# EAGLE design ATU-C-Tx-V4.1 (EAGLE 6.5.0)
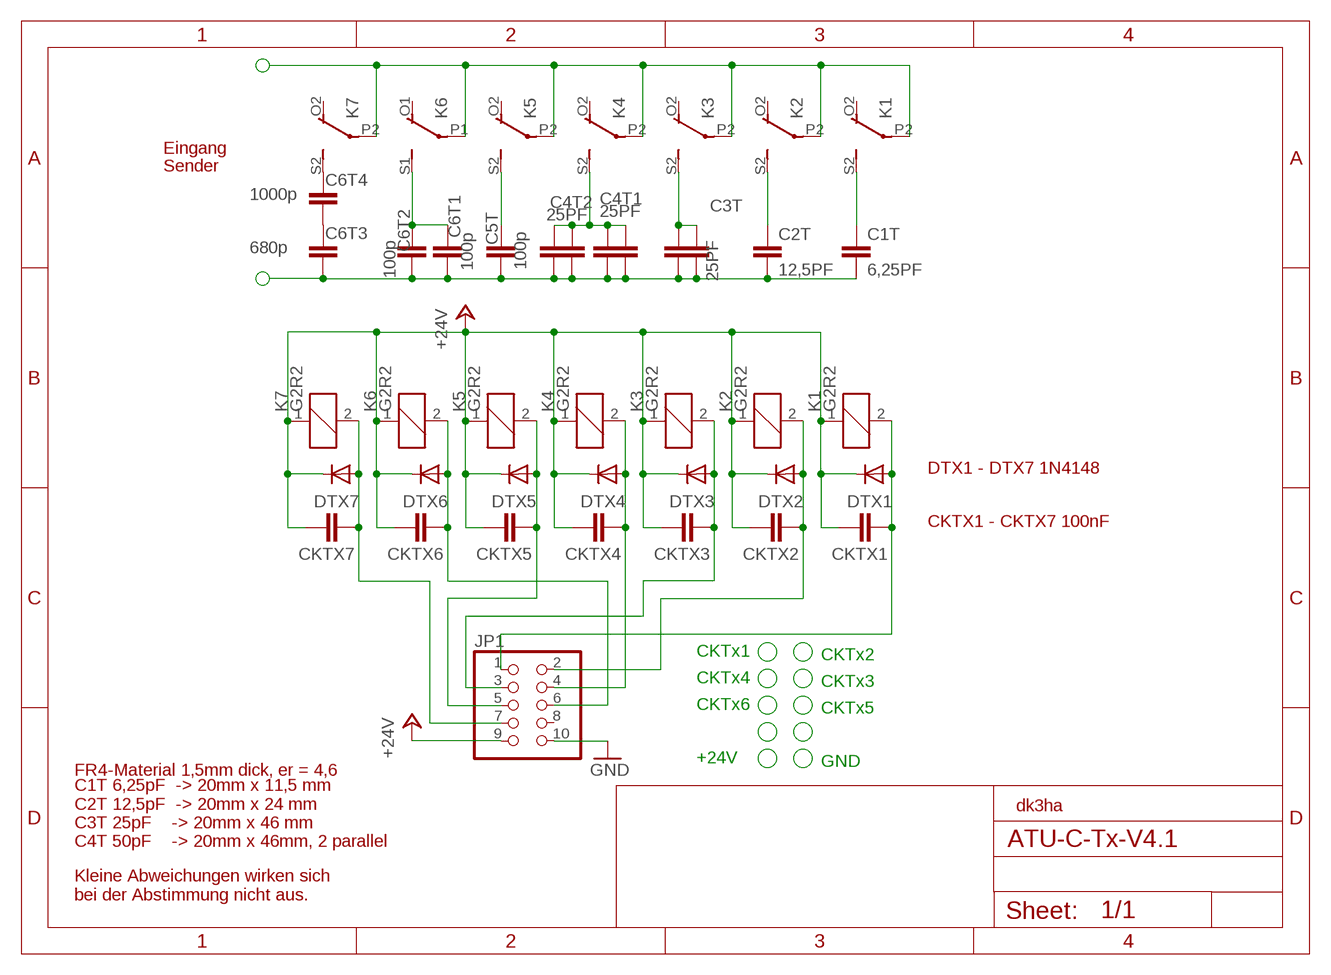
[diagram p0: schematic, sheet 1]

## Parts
C1T  6,25PF  6,25PF-CU-DS-ER4,6-D1,5  [6,25-ERA4,6-DS-1,5]
C2T  12,5PF  12,5PF-CU-DS-ER4,6-D1,5  [12.5-ER4.6-DS-1,5]
C3T  25PF  25PF-CU-DS-ER4,6-D-1,5  [25PF_ER4.6-DS-1,5]
C4T1  25PF  25PF-CU-DS-ER4,6-D-1,5  [25PF_ER4.6-DS-1,5]
C4T2  25PF  25PF-CU-DS-ER4,6-D-1,5  [25PF_ER4.6-DS-1,5]
C5T  100p  C15/5  [C15B5]
C6T1  100p  C15/5  [C15B5]
C6T2  100p  C15/5  [C15B5]
C6T3  680p  C15/5  [C15B5]
C6T4  1000p  C15/5  [C15B5]
CKTX1  C-EUC1206  [C1206]
CKTX2  C-EUC1206  [C1206]
CKTX3  C-EUC1206  [C1206]
CKTX4  C-EUC1206  [C1206]
CKTX5  C-EUC1206  [C1206]
CKTX6  C-EUC1206  [C1206]
CKTX7  C-EUC1206  [C1206]
DTX1  DIODE-MINIMELF  [MINIMELF]
DTX2  DIODE-MINIMELF  [MINIMELF]
DTX3  DIODE-MINIMELF  [MINIMELF]
DTX4  DIODE-MINIMELF  [MINIMELF]
DTX5  DIODE-MINIMELF  [MINIMELF]
DTX6  DIODE-MINIMELF  [MINIMELF]
DTX7  DIODE-MINIMELF  [MINIMELF]
JP1  PINHD-2X5  [2X05]
K1  G2R2  [G2R2]
K2  G2R2  [G2R2]
K3  G2R2  [G2R2]
K4  G2R2  [G2R2]
K5  G2R2  [G2R2]
K6  G2R2  [G2R2]
K7  G2R2  [G2R2]

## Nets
+24V: CKTX1.2 CKTX2.2 CKTX3.2 CKTX4.2 CKTX5.2 CKTX6.2 CKTX7.2 DTX1.C DTX2.C DTX3.C DTX4.C DTX5.C DTX6.C DTX7.C JP1.9 K1.1 K2.1 K3.1 K4.1 K5.1 K6.1 K7.1
GND: JP1.10
LSP7: K1.P2(3:P) K2.P2(3:P) K3.P2(3:P) K4.P2(3:P) K5.P2(3:P) K6.P1(2:P) K7.P2(3:P)
LSP8: C1T.P$2 C2T.P$2 C3T.P$2 C3T.P$4 C4T1.P$2 C4T1.P$4 C4T2.P$2 C4T2.P$4 C5T.2 C6T1.2 C6T2.1 C6T3.1
N$1: CKTX4.1 DTX4.A JP1.4 K4.2
N$2: C4T1.P$1 C4T1.P$3 C4T2.P$1 C4T2.P$3 K4.S2(3:S)
N$3: C6T1.1 C6T2.2 K6.S1(2:S)
N$4: CKTX7.1 DTX7.A JP1.7 K7.2
N$5: C3T.P$1 C3T.P$3 K3.S2(3:S)
N$6: C2T.P$1 K2.S2(3:S)
N$7: C1T.P$1 K1.S2(3:S)
N$8: C5T.1 K5.S2(3:S)
N$9: C6T4.2 K7.S2(3:S)
N$10: C6T3.2 C6T4.1
N$E1: CKTX1.1 DTX1.A JP1.1 K1.2
N$E2: CKTX2.1 DTX2.A JP1.2 K2.2
N$E3: CKTX3.1 DTX3.A JP1.3 K3.2
N$E5: CKTX5.1 DTX5.A JP1.5 K5.2
N$E6: CKTX6.1 DTX6.A JP1.6 K6.2
Unconnected: JP1.8 K1.O1(2:O) K1.O2(3:O) K1.P1(2:P) K1.S1(2:S) K2.O1(2:O) K2.O2(3:O) K2.P1(2:P) K2.S1(2:S) K3.O1(2:O) K3.O2(3:O) K3.P1(2:P) K3.S1(2:S) K4.O1(2:O) K4.O2(3:O) K4.P1(2:P) K4.S1(2:S) K5.O1(2:O) K5.O2(3:O) K5.P1(2:P) K5.S1(2:S) K6.O1(2:O) K6.O2(3:O) K6.P2(3:P) K6.S2(3:S) K7.O1(2:O) K7.O2(3:O) K7.P1(2:P) K7.S1(2:S)

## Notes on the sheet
- Eingang
- Sender
- DTX1 - DTX7 1N4148
- CKTX1 - CKTX7 100nF
- CKTx1 | CKTx2
- CKTx4 | CKTx3
- CKTx6 | CKTx5
- +24V | GND
- FR4-Material 1,5mm dick, er = 4,6
- dk3ha
- C1T 6,25pF  -> 20mm x 11,5 mm
  C2T 12,5pF  -> 20mm x 24 mm
  C3T 25pF    -> 20mm x 46 mm
  C4T 50pF    -> 20mm x 46mm, 2 parallel
- Kleine Abweichungen wirken sich
  bei der Abstimmung nicht aus.

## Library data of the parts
C1T = dk3ha-2020:6,25PF-CU-DS-ER4,6-D1,5: C doppelseitig Cu, d=1,5mm, Epoxy er=4,6 (Bungard), 25 pF, Maße 18,7mm x 13mm
C2T = dk3ha-2020:12,5PF-CU-DS-ER4,6-D1,5: C doppelseitig Cu, d=1,5mm, Epoxy er=4,6 (Bungard), 25 pF, Maße 27,5mm x 18mm
C3T C4T1 C4T2 = dk3ha-2020:25PF-CU-DS-ER4,6-D-1,5: C doppelseitig Cu, d=1,5mm, Epoxy er=4,6 (Bungard), 25 pF, Maße 49,4mm x 18mm
C5T C6T1-C6T4 = capacitor-wima:C: CAPACITOR
CKTX1-CKTX7 = rcl:C-EU: CAPACITOR, European symbol
DTX1-DTX7 = diode:DIODE-: DIODE
JP1 = pinhead+:PINHD-2X5: PIN HEADER
K1-K7 = relay:G2R2: RELAY 2 x switch, Omron; MF: OMRON COMPONENTS USA; MPN: G2R-2-DC6; OC_FARNELL: unknown; OC_NEWARK: 89C5317

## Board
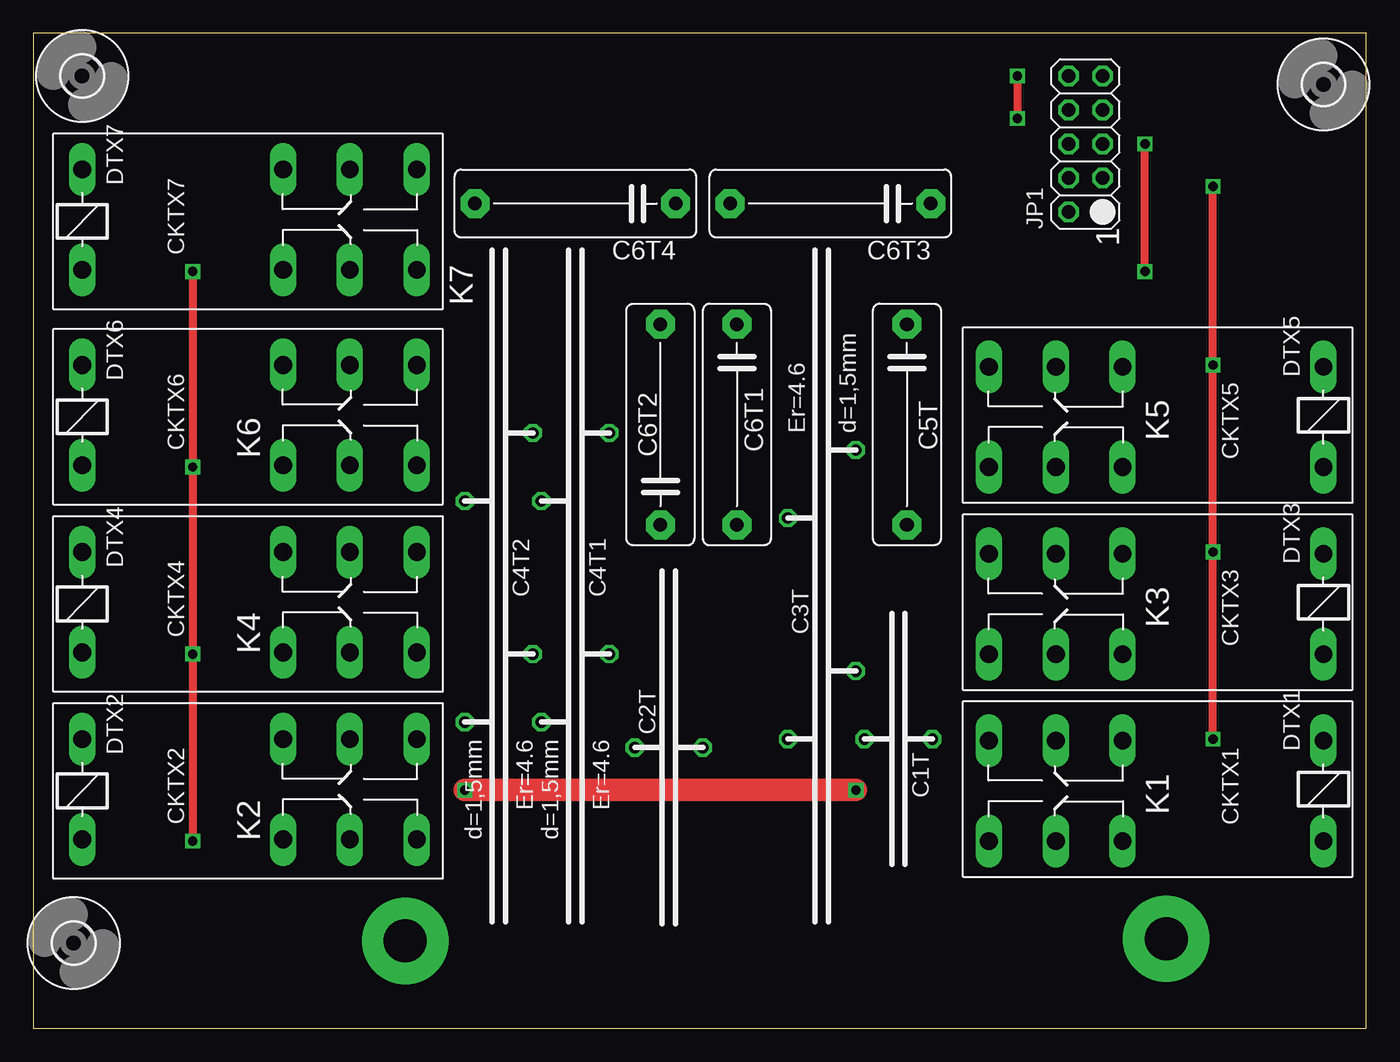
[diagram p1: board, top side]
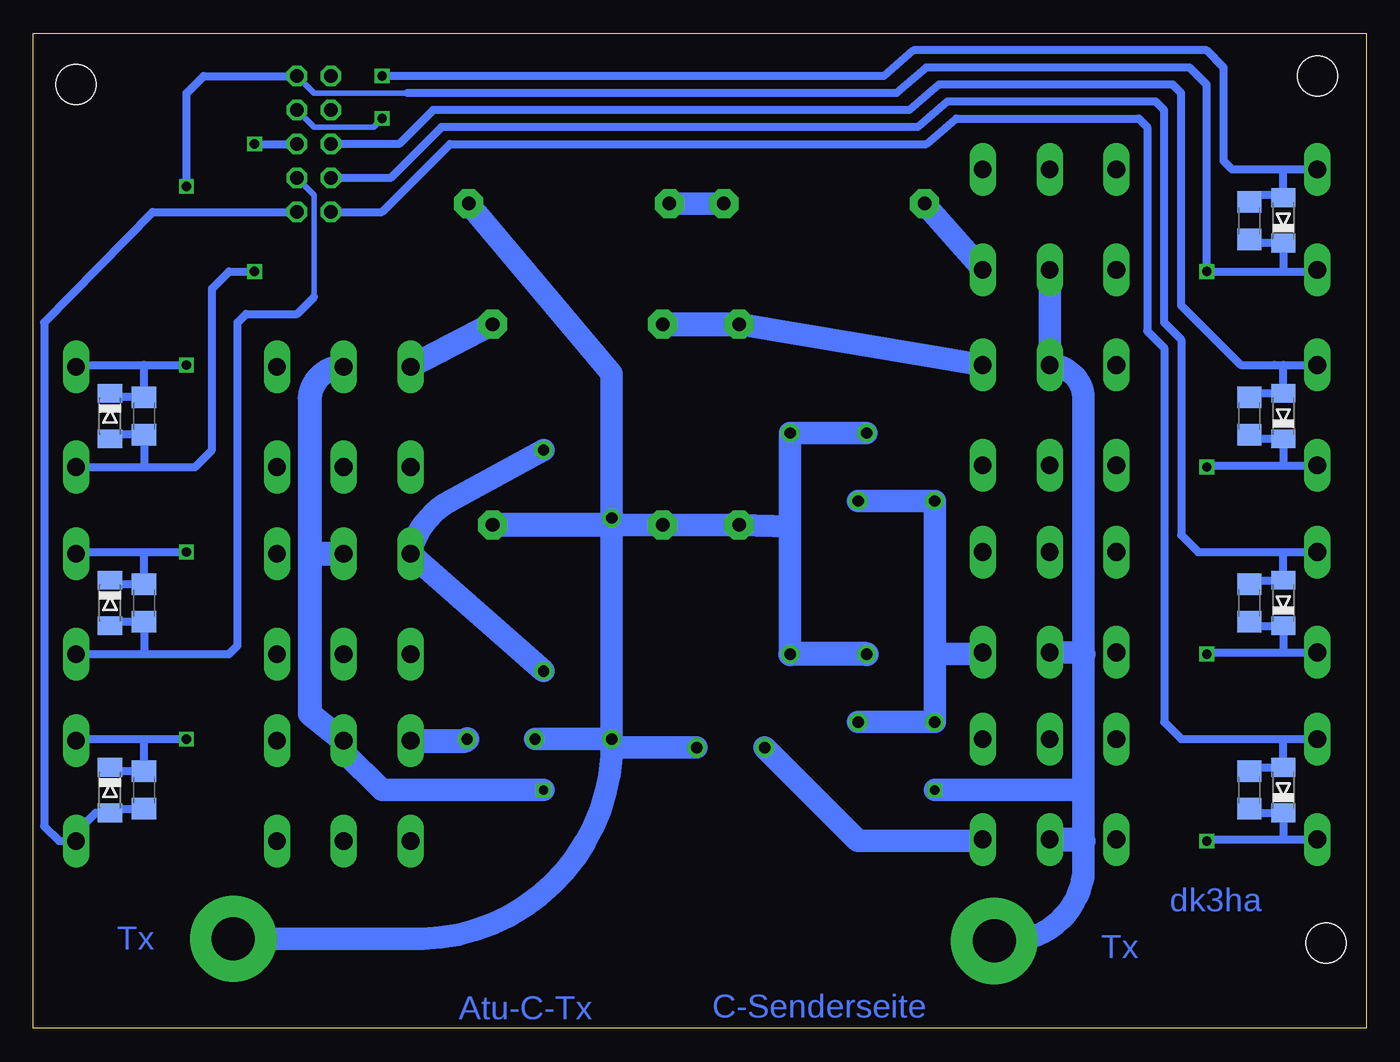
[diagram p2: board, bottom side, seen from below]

Size 99.52 x 74.3 mm. Coordinates in mm from the lower left corner, seen from the top.
Outline: 99.52,0 99.52,74.3 0,74.3 0,0 99.52,0
Copper layers (1*16): Top 0.035mm / dielectric 1.5mm / Bottom 0.035mm
Design rules "default": minimum track width 10mil, minimum drill 24mil, track to track 8mil, track to pad 8mil, pad to pad 8mil, via to via 8mil, smd to smd 8mil, copper to edge 40mil, drill to drill 8mil, minimum pad ring 10mil, minimum via ring 8mil, stop-mask expansion 4mil, vias tented up to drill 0mil, thermal gap 10mil

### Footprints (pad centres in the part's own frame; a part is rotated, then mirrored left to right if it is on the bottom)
6,25-ERA4,6-DS-1,5 = drill 0.85 octagon: P$1 -2.54,0; P$2 2.54,0
12.5-ER4.6-DS-1,5 = drill 0.85 octagon: P$1 -2.54,0; P$2 2.54,0
25PF_ER4.6-DS-1,5 = drill 0.85 pad 1.27 octagon: P$1 0,0; P$2 -5.08,-5.08 | drill 0.85 octagon: P$3 0,-16.51; P$4 -5.08,-21.59
C15B5 = drill 1.016 pad 2.159 octagon: 1 -7.493,0; 2 7.493,0
C1206 = smd 1.6 x 1.8: 1 -1.4,0; 2 1.4,0
MINIMELF = smd 1.4 x 1.8: A 1.7,0; C -1.7,0
2X05 = drill 1.016 octagon: 1 -5.08,-1.27; 2 -5.08,1.27; 3 -2.54,-1.27; 4 -2.54,1.27; 5 0,-1.27; 6 0,1.27; 7 2.54,-1.27; 8 2.54,1.27; 9 5.08,-1.27; 10 5.08,1.27
G2R2 = drill 1.321 long: 1 -2.54,-3.683; 2 -2.54,3.81; O1 12.471,3.81; O2 12.471,-3.683; P1 17.45,3.81; P2 17.45,-3.683; S1 22.454,3.81; S2 22.454,-3.683
3,0 = hole 3: 0,0

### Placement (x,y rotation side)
C1T  64.6,21.59 180 top
C2T  47.45,20.95 0 top
C3T  61.42,43.18 0 top
C4T1  37.93,22.86 180 top
C4T2  32.21,22.86 180 top
C5T  65.23,45.09 270 top
C6T1  52.53,45.09 270 top
C6T2  46.82,45.09 90 top
C6T3  59.52,61.59 180 top
C6T4  40.47,61.59 180 top
CKTX1  91.27,17.78 90 bottom
CKTX2  8.72,17.78 270 bottom
CKTX3  91.27,31.75 90 bottom
CKTX4  8.72,31.75 270 bottom
CKTX5  91.27,45.72 90 bottom
CKTX6  8.72,45.72 270 bottom
CKTX7  8.72,60.33 270 bottom
DTX1  93.81,17.78 270 bottom
DTX2  6.18,17.78 90 bottom
DTX3  93.81,31.75 270 bottom
DTX4  6.18,31.75 90 bottom
DTX5  93.81,45.72 270 bottom
DTX6  6.18,45.72 90 bottom
DTX7  6.18,60.33 90 bottom
JP1  78.57,66.04 90 top
K1  93.81,17.78 180 top
K2  6.18,17.78 0 top
K3  93.81,31.75 180 top
K4  6.18,31.75 0 top
K5  93.81,45.72 180 top
K6  6.18,45.72 0 top
K7  6.18,60.33 0 top
U$1  [3,0]  3.64,71.12 90 top
U$2  [3,0]  96.35,70.48 90 top
U$3  [3,0]  3,6.35 90 top

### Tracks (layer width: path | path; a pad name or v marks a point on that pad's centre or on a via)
+24V  (via drill 0.7)
  Top 0.61: v88.09,21.59 v88.09,35.56 v88.09,49.53 v88.09,62.87 | v11.89,56.52 v11.89,41.91 v11.89,27.94 v11.89,13.97
  Bottom 0.406: 71.58,69.85 78.57,69.85 JP1.9
  Bottom 0.61: v11.89,13.97 11.89,14.1 6.18,14.1 | 6.18,14.1 K2.1 | v11.89,27.94 11.89,28.07 6.18,28.07 | 6.18,28.07 K4.1 | v11.89,41.91 11.89,42.04 6.18,42.04 | 6.18,42.04 K6.1 | CKTX2.2 8.72,16.08 DTX2.C 6.18,14.1 | CKTX4.2 8.72,30.05 DTX4.C 6.18,28.07 | CKTX6.2 8.72,44.02 DTX6.C 6.18,42.04 | K1.1 96.35,21.59 91.27,21.59 | 91.27,21.59 v88.09,21.59 | K3.1 96.35,35.56 91.27,35.56 | 91.27,35.56 v88.09,35.56 | K5.1 96.35,49.53 91.27,49.53 | 91.27,49.53 v88.09,49.53 | CKTX7.2 8.42,58.62 DTX7.C 6.18,56.52 | 6.18,56.52 v11.89,56.52 11.89,70.48 13.16,71.75 32.85,71.75 35.07,69.85 71.58,69.85 | 6.18,56.52 3.77,56.52 K7.1 | v88.09,62.87 88.09,69.85 86.82,71.12 JP1.9 | 91.27,35.56 CKTX3.2 93.51,33.15 DTX3.C | 91.27,49.53 CKTX5.2 93.51,47.12 DTX5.C | 91.27,21.59 CKTX1.2 93.51,19.18 DTX1.C
  Bottom 0.813: K6.1 3.64,41.91
LSP7  (via drill 0.7, 3.2 pad 6.45)
  Top 1.676: v61.42,17.78 v32.21,17.78
  Bottom 1.676: 21.1,17.78 21.1,13.97 21.1,11.43 arc90 v27.77,6.51 | 21.1,17.78 21.1,27.94 21.1,47 arc-90 K6.P1 K7.P2 | K4.P2 21.23,28.07 | v61.42,17.78 73.49,17.78 76.36,20.65 K1.P2 | v32.21,17.78 21.1,17.78
  Bottom 1.778: K2.P2 21.23,14.1 21.1,13.97 | 21.23,28.07 21.1,27.94 | 78.89,35.56 78.89,46.88 arc90 K5.P2 | 78.89,35.56 78.89,23.5 78.76,23.37 K1.P2 | K3.P2 78.76,35.43 78.89,35.56
LSP8  (via drill 3.2 pad 6.45)
  Bottom 1.676: C4T1.P$2 43.01,37.47 | 43.01,37.47 C4T1.P$4 C4T2.P$4 | C3T.P$4 56.34,37.59 C3T.P$2 56.34,48.9 C6T3.1 | v84.6,6.67 70.47,6.67 arc-90 C3T.P$4 | C2T.P$2 56.34,20.95 C3T.P$4 | C1T.P$2 C3T.P$4 | 43.01,37.47 C6T2.1 C6T1.2 56.98,37.59
  Bottom 1.778: C4T2.P$2 C4T1.P$2 | 56.34,37.59 56.98,37.59 C5T.2
N$1
  Bottom 0.61: 6.18,35.56 12.53,35.56 13.8,36.83 13.8,51.44 15.07,52.7 15.07,68.58 15.7,69.22 31.26,69.22 33.48,67.31 69.04,67.31 72.85,63.5 JP1.4 | 6.18,35.56 K4.2 | CKTX4.1 8.72,33.45 DTX4.A 6.18,35.56
N$2
  Bottom 1.676: C4T1.P$1 C4T2.P$1 32.21,27.94 | 32.21,27.94 C4T2.P$3 C4T1.P$3 | 28.76,27.94 32.21,27.94
  Bottom 1.778: 28.76,27.94 K4.S2
N$3
  Bottom 1.676: C6T2.2 K6.S1
  Bottom 1.778: C6T1.1 C6T2.2
N$4  (via drill 0.7 pad 0.81)
  Top 0.61: v73.49,71.12 v73.49,67.94
  Bottom 0.406: v73.49,67.94 74.12,67.31 78.57,67.31 JP1.7
  Bottom 0.61: 8.42,62.02 CKTX7.1 8.72,62.23 6.18,62.23 DTX7.A 6.18,64.14 | K7.2 6.18,64.14 | 6.18,64.14 9.99,64.14 10.62,64.77 10.62,71.75 11.89,73.03 33.8,73.03 36.02,71.12 v73.49,71.12
N$5
  Bottom 1.676: C3T.P$3 K3.S2 arc49 68.41,39.37 C3T.P$1
N$6
  Bottom 1.676: C2T.P$1 37.93,13.97 28.76,13.97 K2.S2
N$7
  Bottom 1.778: K1.S2 67.27,21.46 C1T.P$1
N$8
  Bottom 1.778: C5T.1 K5.S2
N$9
  Bottom 1.676: C6T4.2 K7.S2
N$10
  Bottom 1.676: C6T4.1 C6T3.2
N$E1
  Bottom 0.61: JP1.1 90.63,60.96 98.73,52.7 98.73,15.08 97.62,13.97 K1.2 96.35,14.61 94.87,16.08 DTX1.A 93.81,16.38 CKTX1.1
N$E2
  Bottom 0.61: 6.18,21.59 13.8,21.59 15.07,22.86 15.07,50.8 16.34,52.07 16.34,67.31 16.97,67.94 30.63,67.94 32.85,66.04 68.41,66.04 73.49,60.96 JP1.2 | 6.18,21.59 K2.2 | CKTX2.1 8.72,19.48 DTX2.A 6.18,21.59
N$E3
  Bottom 0.406: 78.57,54.61 78.57,62.23 JP1.3
  Bottom 0.61: K3.2 91.27,27.94 | 91.27,27.94 84.92,27.94 84.28,28.57 84.28,52.7 83.65,53.34 79.84,53.34 78.57,54.61 | 91.27,27.94 CKTX3.1 93.51,30.35 DTX3.A
N$E5  (via drill 0.7 pad 0.81)
  Top 0.61: v83.01,56.52 v83.01,66.04
  Bottom 0.61: K5.2 91.27,41.91 | 91.27,41.91 87.46,41.91 86.19,43.18 86.19,55.24 84.92,56.52 v83.01,56.52 | v83.01,66.04 JP1.5 | 91.27,41.91 CKTX5.1 93.51,44.32 DTX5.A
N$E6
  Bottom 0.406: 8.72,49.53 6.81,49.53
  Bottom 0.61: 6.18,49.53 6.81,49.53 9.35,49.53 13.8,53.98 13.8,69.85 14.43,70.48 31.9,70.48 34.12,68.58 69.68,68.58 72.22,66.04 JP1.6 | 6.18,49.53 K6.2 | CKTX6.1 8.72,47.42 DTX6.A 6.18,49.53

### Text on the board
Bottom: dk3ha | Tx | Tx | C-Senderseite | Atu-C-Tx
tPlace: 1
